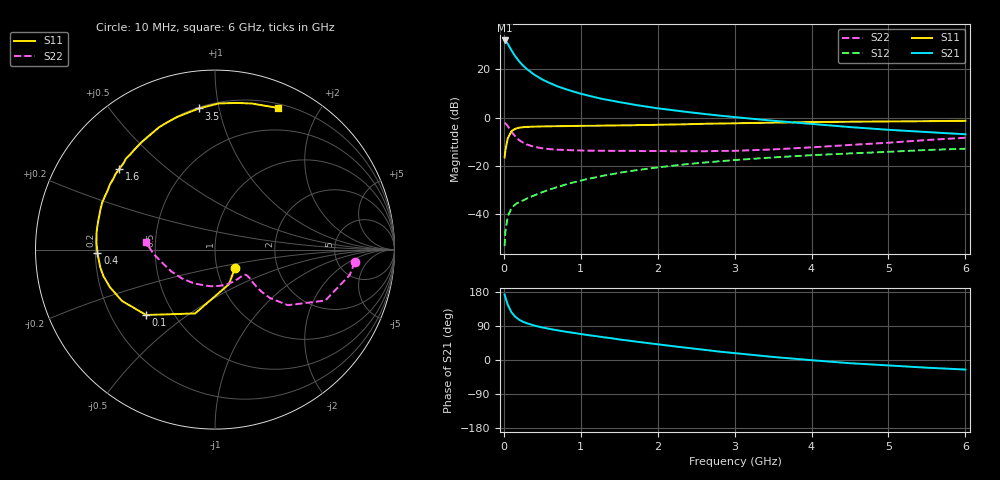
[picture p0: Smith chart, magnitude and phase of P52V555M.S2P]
! SIEMENS Small Signal Semiconductors
! BFP183
! Si NPN RF Bipolar Junction Transistor in SOT143
! VCE = 2.5 V  IC = 55 mA
! Common Emitter S-Parameters:  March  1996
# GHz  S  MA  R  50
!  f  S11  S21  S12  S22
! GHz  MAG  ANG  MAG  ANG  MAG  ANG  MAG  ANG
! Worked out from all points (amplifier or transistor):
!   36 points, 10 MHz to 6 GHz, reference 50 ohm
!   highest |S21| = 32.0 dB at 10 MHz (marker M1)
!   |S21| within 3 dB of that: start of sweep to 79.72 MHz
!   unconditionally stable (mu >= 1): start of sweep to 25.64 MHz; 221.9 MHz to end of sweep
!   at 250 MHz: K = 1.08, MAG = 26.2 dB, |S12| = -34.2 dB
!   at 1.4 GHz: K = 1.58, MAG = 10.8 dB, |S12| = -23.4 dB
!   at 6 GHz: K = 1.21, MAG = 0.2 dB, |S12| = -12.8 dB
!   S11 on the Smith chart (normalised r, x): 10 MHz: 1.22, -0.25; 100 MHz: 0.35, -0.36; 400 MHz: 0.21, -0.02; 1.6 GHz: 0.20, +0.35; 3.5 GHz: 0.21, +0.87; 6 GHz: 0.24, +1.51
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0.01  0.1511 -42.2  39.77 172.7  0.0022 67.1  0.7815 -5.1
0.02  0.2082 -68.2  39.18 165.5  0.0044 65.8  0.7639 -10.7
0.05  0.3725 -107.3  34.15 146.3  0.009 63.6  0.6767 -24.8
0.1  0.5293 -136.5  24.68 125.6  0.0136 51.8  0.5112 -37.3
0.15  0.5919 -151.1  18.6 113.8  0.0162 48.7  0.4071 -41.4
0.2  0.6221 -160.4  14.62 106.2  0.0181 48.5  0.3441 -42.2
0.25  0.6389 -166.6  11.98 100.9  0.0194 49.5  0.3051 -41.7
0.3  0.6468 -171.2  10.15 97.0  0.0214 50.7  0.2787 -40.9
0.4  0.655 -178.2  7.715 90.6  0.0249 55.8  0.2496 -39.5
0.5  0.6619 176.5  6.18 85.9  0.0288 57.1  0.2335 -39.0
0.6  0.6666 171.6  5.212 81.8  0.033 58.8  0.2238 -39.2
0.7  0.6689 167.9  4.451 78.2  0.0369 59.9  0.2186 -39.9
0.9  0.6761 161.0  3.502 71.8  0.0458 61.2  0.2126 -42.6
1.1  0.6818 154.1  2.869 65.5  0.0547 61.2  0.2087 -46.3
1.3  0.6888 148.4  2.419 59.9  0.0636 60.6  0.2076 -50.9
1.6  0.698 139.7  1.985 51.8  0.0766 58.9  0.2069 -58.0
2.2  0.7252 124.1  1.433 36.4  0.102 53.6  0.203 -75.9
2.8  0.758 110.1  1.11 22.2  0.1257 47.5  0.2055 -96.4
3.5  0.7915 96.5  0.867 8.1  0.1511 40.6  0.2212 -121.4
4.5  0.8263 81.5  0.641 -8.5  0.1826 30.4  0.2736 -154.0
5.5  0.8491 70.6  0.506 -20.3  0.2154 21.1  0.346 -176.6
6  0.8642 66.0  0.455 -25.2  0.2283 15.9  0.3856 174.0
